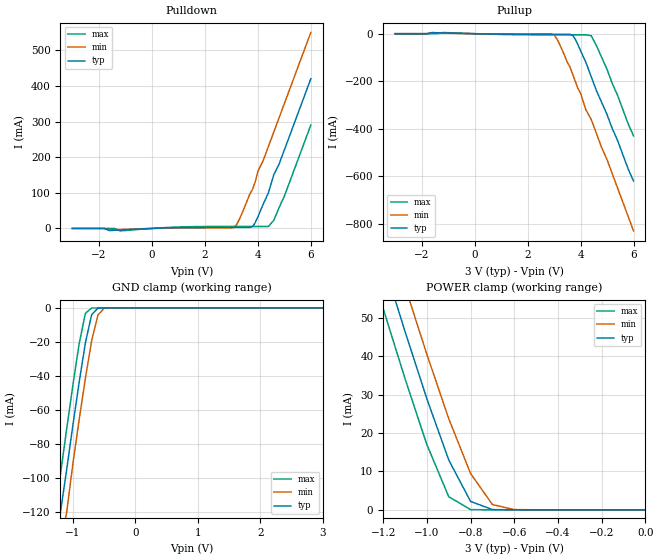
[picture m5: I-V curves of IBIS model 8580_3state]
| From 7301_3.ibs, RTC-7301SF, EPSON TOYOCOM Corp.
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|   Model   8580_3state
[Model]   8580_3state
Model_type   3-state
Polarity   Inverting
C_comp   8.00pF   8.00pF   8.00pF
[Temperature Range]   25   85   -40
[Voltage Range]   3.00V   2.40V   3.60V
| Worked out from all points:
|   slope of the pulldown table from 0 to 0.45 V, typ, clamps not added: 346 ohm
|   slope of the pullup table from 0 to 0.45 V, typ, clamps not added: 474 ohm
|   GND clamp passes 1 mA (typ) near -0.62 V on its own axis
|   POWER clamp passes 1 mA (typ) near -0.74 V on its own axis
[Pulldown]
|   voltage   I(typ)   I(min)   I(max)
-3V       0A         0A         0A
-1.4V     -5.09mA    -3.39mA    0A
-1.2V     -4.49mA    -2.98mA    -6.79mA
3.1V      2.89mA     2.77mA     5.47mA
3.3V      2.9mA      25.15mA    5.48mA
3.8V      5.09mA     110mA      5.49mA
3.9V      15.91mA    130mA      5.49mA
4V        31.8mA     160mA      5.49mA
4.4V      100mA      230mA      5.55mA
4.6V      150mA      270mA      22.48mA
5V        220mA      350mA      90.27mA
6V        420mA      550mA      290mA
[Pullup]
|   voltage   I(typ)   I(min)   I(max)
-3V       0A         0A         0A
-1.2V     3.25mA     2.18mA     5.03mA
3V        -2.47mA    -5.37mA    -4.82mA
3.2V      -2.48mA    -42.34mA   -4.84mA
3.7V      -6.45mA    -170mA     -4.87mA
3.9V      -46.01mA   -230mA     -4.88mA
4V        -71.24mA   -250mA     -4.89mA
4.2V      -120mA     -320mA     -4.9mA
4.4V      -180mA     -360mA     -8.08mA
4.6V      -240mA     -420mA     -50mA
5V        -340mA     -530mA     -150mA
6V        -620mA     -830mA     -430mA
[GND_clamp]
|   voltage   I(typ)   I(min)   I(max)
-3V       -620mA     -650mA     -600mA
-1.3V     -150mA     -170mA     -120mA
-1.2V     -120mA     -140mA     -97.79mA
-1.1V     -94.94mA   -120mA     -71.05mA
-1V       -68.74mA   -91.25mA   -45.09mA
-900mV    -43.52mA   -65.59mA   -20.92mA
-800mV    -20.48mA   -41.13mA   -3.17mA
-700mV    -3.96mA    -19.25mA   -37.79uA
-600mV    -140uA     -4.17mA    -260nA
-500mV    -2.83uA    -250uA     -1.81nA
3V        3.01pA     66.2uA     2.4pA
[POWER_clamp]
|   voltage   I(typ)   I(min)   I(max)
-3V       420mA      430mA      400mA
-1.3V     83.45mA    95.19mA    71.21mA
-1.2V     64.75mA    76.53mA    52.43mA
-1.1V     46.44mA    58.21mA    34.17mA
-1V       28.9mA     40.47mA    16.98mA
-900mV    13mA       23.75mA    3.42mA
-800mV    2.18mA     9.45mA     54.44uA
-700mV    67.16uA    1.37mA     380nA
-600mV    1.39uA     66.2uA     2.63nA
0V        3.01pA     26.51pA    3.6pA
[Ramp]
|variable   typ   min   max
dV/dt_r   1.65/1.36n   1.25/2.23n   2.05/0.80n
dV/dt_f   1.69/1.36n   1.30/2.22n   2.08/0.92n
R_load = 5.00k
|   End   [Model]   8580_3state
